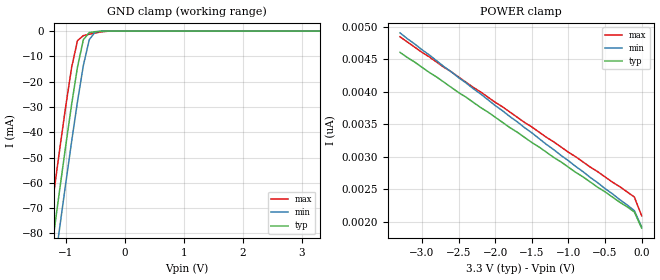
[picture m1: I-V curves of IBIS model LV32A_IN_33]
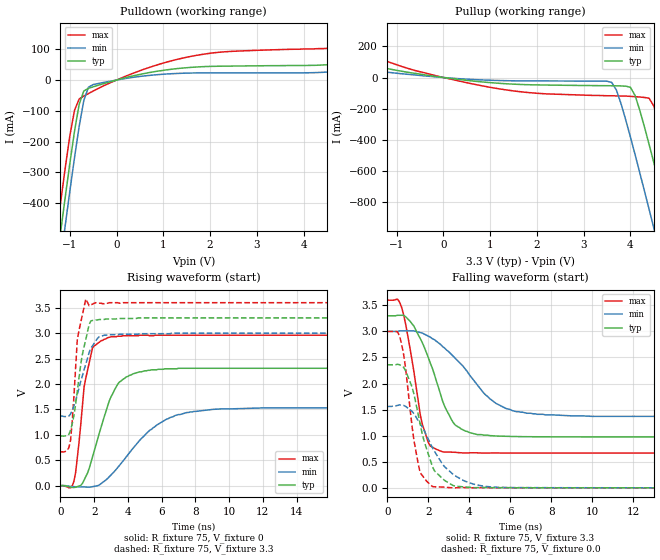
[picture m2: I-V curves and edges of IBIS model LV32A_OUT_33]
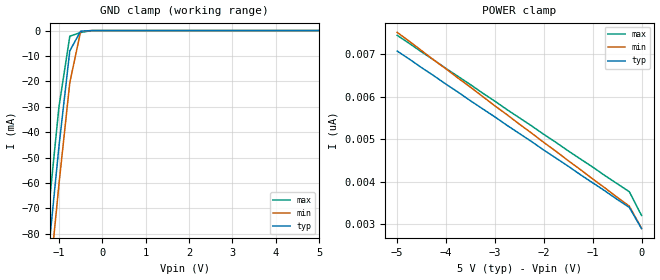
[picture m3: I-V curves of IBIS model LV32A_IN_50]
| TEXAS INSTRUMENTS INCORPORATED
| Standard Linear and Logic Group
| IBIS Model of SN74LV32A
| QUADRUPLE 2-INPUT POSITIVE-NOR GATE
| SOIC 14-pin (D), SOP 14-pin (NS), SSOP 14-pin (DB), TSSOP 14-pin (PW)
| and TVSOP 14-pin (DGV) Package
[IBIS Ver]   3.2
[Comment Char]  |_char
[File Name]   lv32a.ibs
[File Rev]   2.0 H_die
[Date]   May 26, 2000
[Source]   Data created from HSPICE simulations at TI-SLL.
[Notes]   The following is an IBIS list for the LV32A.
|   Please contact sllibis@ti.com with questions and
|   comments concerning SLL IBIS models.
|   The warning about AC Rising Endpoint might be reported,
|   but it is due to HSPICE issue and negligible.
[Disclaimer] Property of Texas Instruments Incorporated.  Unauthorized
   reproduction and/or distribution is strictly prohibited.
   This product is protected under copyright law.
   Created 2000, (C) Copyright 2000, Texas Instruments Inc.,
   All Rights Reserved.
   UNLESS THERE IS A SIGNED, WRITTEN AGREEMENT TO THE
   CONTRARY, TEXAS INSTRUMENTS () IS PROVIDING THE IBIS
   MODELS  AND WITHOUT ANY WARRANTY, EXPRESSED OR
   IMPLIED.  TI assumes no liability for:
   1) the accuracy of the IBIS models provided to your
   company;
   2) the proper functioning of these IBIS Models in your
   design or for any resulting applications; or
   3) infringement of patents, copyrights or intellectual
   property rights resulting from your use of these IBIS
   models.
   TI provides IBIS Models as a service to our customers.
   You and your company shall not distribute, sell or give
   these models to anyone else without prior written
   permission from TI.
   TI reserves the right to make changes to our products or
   to discontinue any semiconductor product or service
   without notice, and advises our customers to obtain the
   latest version of relevant information to verify, before
   placing orders, that the information being relied on is
   current.
   Please be aware that your receipt and use of the IBIS
   information provided shall serve as acceptance of these
   terms and conditions.  If you do not accept these terms,
   you should return or destroy the IBIS models and any
   other accompanying information immediately.
|   Component LV32A_D
[Component]   LV32A_D
[Manufacturer]  Texas Instruments, Inc.
[Package]
|   typ   min   max
R_pkg   0.031   0.028   0.034
L_pkg   3.109nH   2.462nH   3.889nH
C_pkg   0.473pF   0.363pF   0.628pF
[Pin]   signal_name   model_name   R_pin   L_pin   C_pin
1   1A   LV32A_IN   0.033   3.854nH   0.622pF
2   1B   LV32A_IN   0.032   3.188nH   0.473pF
3   1Y   LV32A_OUT   0.028   2.462nH   0.377pF
4   2A   LV32A_IN   0.031   2.596nH   0.363pF
5   2B   LV32A_IN   0.028   2.521nH   0.372pF
6   2Y   LV32A_OUT   0.034   3.250nH   0.476pF
7   GND   GND   0.034   3.889nH   0.628pF
8   3Y   LV32A_OUT   0.034   3.889nH   0.628pF
9   3A   LV32A_IN   0.034   3.250nH   0.476pF
10   3B   LV32A_IN   0.028   2.521nH   0.372pF
11   4Y   LV32A_OUT   0.031   2.596nH   0.364pF
12   4A   LV32A_IN   0.028   2.462nH   0.377pF
13   4B   LV32A_IN   0.032   3.188nH   0.473pF
14   VCC   POWER   0.033   3.854nH   0.622pF
|   Component LV32A_NS
[Component]   LV32A_NS
[Manufacturer]  Texas Instruments, Inc.
[Package]
|   typ   min   max
R_pkg   0.045   0.039   0.054
L_pkg   3.796nH   2.561nH   4.952nH
C_pkg   0.528pF   0.288pF   0.710pF
[Pin]   signal_name   model_name   R_pin   L_pin   C_pin
1   1A   LV32A_IN   0.047   4.867nH   0.706pF
2   1B   LV32A_IN   0.051   4.083nH   0.592pF
3   1Y   LV32A_OUT   0.041   2.915nH   0.376pF
4   2A   LV32A_IN   0.039   2.561nH   0.288pF
5   2B   LV32A_IN   0.041   3.101nH   0.430pF
6   2Y   LV32A_OUT   0.047   4.047nH   0.589pF
7   GND   GND   0.051   4.909nH   0.700pF
8   3Y   LV32A_OUT   0.045   4.784nH   0.694pF
9   3A   LV32A_IN   0.054   4.176nH   0.597pF
10   3B   LV32A_IN   0.039   3.287nH   0.449pF
11   4Y   LV32A_OUT   0.039   2.586nH   0.294pF
12   4A   LV32A_IN   0.040   2.802nH   0.371pF
13   4B   LV32A_IN   0.049   4.080nH   0.593pF
14   VCC   POWER   0.052   4.952nH   0.710pF
|   Component LV32A_DB
[Component]   LV32A_DB
[Manufacturer]  Texas Instruments, Inc.
[Package]
|   typ   min   max
R_pkg   0.044   0.041   0.046
L_pkg   3.551nH   3.258nH   3.927nH
C_pkg   0.402pF   0.360pF   0.421pF
[Pin]   signal_name   model_name   R_pin   L_pin   C_pin
1   1A   LV32A_IN   0.046   3.927nH   0.408pF
2   1B   LV32A_IN   0.044   3.587nH   0.421pF
3   1Y   LV32A_OUT   0.041   3.289nH   0.398pF
4   2A   LV32A_IN   0.042   3.258nH   0.360pF
5   2B   LV32A_IN   0.041   3.286nH   0.403pF
6   2Y   LV32A_OUT   0.044   3.586nH   0.421pF
7   GND   GND   0.046   3.927nH   0.408pF
8   3Y   LV32A_OUT   0.046   3.927nH   0.408pF
9   3A   LV32A_IN   0.044   3.586nH   0.421pF
10   3B   LV32A_IN   0.041   3.286nH   0.403pF
11   4Y   LV32A_OUT   0.043   3.258nH   0.360pF
12   4A   LV32A_IN   0.041   3.289nH   0.398pF
13   4B   LV32A_IN   0.044   3.587nH   0.421pF
14   VCC   POWER   0.046   3.927nH   0.408pF
|   Component LV32A_PW
[Component]   LV32A_PW
[Manufacturer]  Texas Instruments, Inc.
[Package]
|   typ   min   max
R_pkg   0.032   0.029   0.035
L_pkg   2.378nH   2.170nH   2.680nH
C_pkg   0.314pF   0.270pF   0.335pF
[Pin]   signal_name   model_name   R_pin   L_pin   C_pin
1   1A   LV32A_IN   0.033   2.618nH   0.330pF
2   1B   LV32A_IN   0.031   2.313nH   0.317pF
3   1Y   LV32A_OUT   0.030   2.310nH   0.314pF
4   2A   LV32A_IN   0.031   2.173nH   0.272pF
5   2B   LV32A_IN   0.030   2.204nH   0.309pF
6   2Y   LV32A_OUT   0.032   2.315nH   0.317pF
7   GND   GND   0.035   2.680nH   0.335pF
8   3Y   LV32A_OUT   0.033   2.640nH   0.333pF
9   3A   LV32A_IN   0.034   2.347nH   0.319pF
10   3B   LV32A_IN   0.029   2.277nH   0.313pF
11   4Y   LV32A_OUT   0.031   2.170nH   0.270pF
12   4A   LV32A_IN   0.031   2.244nH   0.311pF
13   4B   LV32A_IN   0.033   2.343nH   0.321pF
14   VCC   POWER   0.035   2.657nH   0.332pF
|   Component LV32A_DGV
[Component]   LV32A_DGV
[Manufacturer]  Texas Instruments, Inc.
[Package]
|   typ   min   max
R_pkg   0.035   0.020   0.045
L_pkg   2.499nH   2.077nH   2.966nH
C_pkg   0.361pF   0.305pF   0.416pF
[Pin]   signal_name   model_name   R_pin   L_pin   C_pin
1   1A   LV32A_IN   0.027   2.717nH   0.373pF
2   1B   LV32A_IN   0.037   2.434nH   0.398pF
3   1Y   LV32A_OUT   0.034   2.200nH   0.316pF
4   2A   LV32A_IN   0.020   2.077nH   0.309pF
5   2B   LV32A_IN   0.030   2.147nH   0.305pF
6   2Y   LV32A_OUT   0.042   2.580nH   0.408pF
7   GND   GND   0.039   2.921nH   0.385pF
8   3Y   LV32A_OUT   0.033   2.841nH   0.380pF
9   3A   LV32A_IN   0.042   2.611nH   0.410pF
10   3B   LV32A_IN   0.038   2.331nH   0.329pF
11   4Y   LV32A_OUT   0.026   2.223nH   0.319pF
12   4A   LV32A_IN   0.034   2.259nH   0.313pF
13   4B   LV32A_IN   0.045   2.681nH   0.416pF
14   VCC   POWER   0.042   2.966nH   0.386pF
[Model Selector]   LV32A_IN
LV32A_IN_33   3.3-V Vcc Input Model
LV32A_IN_50   5.0-V Vcc Input Model
[Model Selector]   LV32A_OUT
LV32A_OUT_33   3.3-V Vcc Output Model
LV32A_OUT_50   5.0-V Vcc Output Model
| Models and submodels in the file (4): LV32A_IN_33 (Input), LV32A_OUT_33 (Output), LV32A_IN_50 (Input), LV32A_OUT_50 (Output)
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|   Model LV32A_IN_33
[Model]   LV32A_IN_33
Model_type  Input
Polarity   Inverting
Vinl = 0.99
Vinh = 2.31
| variable   typ   min   max
C_comp   1.24pf   0.94pf   1.54pf
[Temperature Range]   25   85   -40
[Voltage Range]   3.3   3.0   3.6
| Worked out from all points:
|   GND clamp passes 1 mA (typ) near -0.61 V on its own axis
[GND Clamp]
|   Voltage   I(typ)   I(min)   I(max)
-3.3V     -460mA     -475mA     -445mA
-1.3V     -97.5mA    -113mA     -81.5mA
-1.2V     -79.9mA    -95mA      -63.9mA
-1.1V     -62.6mA    -77.6mA    -46.7mA
-1V       -45.6mA    -60.5mA    -30mA
-900mV    -29.2mA    -43.9mA    -14.6mA
-800mV    -14.3mA    -28mA      -3.81mA
-700mV    -3.42mA    -13.6mA    -1.78mA
-600mV    -581uA     -3.4mA     -1.25mA
-500mV    -233uA     -353uA     -759uA
-400mV    -58.1uA    -21.9uA    -324uA
3.3V      1.9nA      2.34nA     1.69nA
[POWER Clamp]
|   Voltage   I(typ)   I(min)   I(max)
-3.3V     4.61nA     4.91nA     4.85nA
-3V       4.38nA     4.65nA     4.61nA
-100mV    2.15nA     2.17nA     2.38nA
0V        1.9nA      1.92nA     2.09nA
|   Model LV32A_OUT_33
[Model]   LV32A_OUT_33
Model_type  Output
Polarity   Non-Inverting
Vmeas = 1.65v
Cref = 15pf
| variable   typ   min   max
C_comp   4.62pf   3.47pf   5.77pf
[Temperature Range]   25   85   -40
[Voltage Range]   3.3   3.0   3.6
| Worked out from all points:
|   slope of the pulldown table from 0 to 0.495 V, typ, clamps not added: 27.3 ohm
|   slope of the pullup table from 0 to 0.495 V, typ, clamps not added: 27.2 ohm
|   rising waveform, R_fixture 75, V_fixture 0: 20-80 % time 1.34ns typ, 2.6ns min, 659ps max; typ from 0 V to 2.31 V
|   falling waveform, R_fixture 75, V_fixture 3.3: 20-80 % time 1.31ns typ, 2.23ns min, 735ps max; typ from 3.3 V to 0.976 V
|   rising waveform, R_fixture 75, V_fixture 3.3: 20-80 % time 648ps typ, 847ps min, 383ps max; typ from 0.976 V to 3.3 V
|   falling waveform, R_fixture 75, V_fixture 0.0: 20-80 % time 908ps typ, 1.48ns min, 589ps max; typ from 2.36 V to 0 V
[Pulldown]
|   Voltage   I(typ)   I(min)   I(max)
-3.3V     -3.04A     -3.13A     -2.95A
-1.3V     -615mA     -707mA     -518mA
-1.2V     -498mA     -591mA     -401mA
-1.1V     -383mA     -475mA     -288mA
-900mV    -167mA     -253mA     -98.6mA
-800mV    -79.1mA    -151mA     -61.7mA
-700mV    -35.5mA    -66.4mA    -51.9mA
-600mV    -26.8mA    -23.2mA    -43.9mA
-500mV    -22mA      -14.7mA    -35.8mA
1.6V      41.2mA     22.8mA     77.1mA
4.7V      52.1mA     27.5mA     106mA
6.6V      86.8mA     47.3mA     166mA
[Pullup]
|   Voltage   I(typ)   I(min)   I(max)
-3.3V     166mA      91.1mA     311mA
600mV     -21.6mA    -12.3mA    -39.7mA
3.6V      -52.9mA    -31.5mA    -117mA
3.8V      -54.2mA    -168mA     -119mA
4V        -62.6mA    -381mA     -121mA
4.1V      -115mA     -494mA     -123mA
4.4V      -429mA     -845mA     -133mA
4.5V      -544mA     -964mA     -182mA
4.8V      -899mA     -1.32A     -505mA
4.9V      -1.02A     -1.44A     -622mA
5.2V      -1.38A     -1.81A     -981mA
6.6V      -3.09A     -3.52A     -2.69A
[Ramp]
| variable   typ   min   max
dV/dt_r   1.40E+00/1.34E-09   9.37E-01/2.69E-09   1.78E+00/5.83E-10
dV/dt_f   1.41E+00/1.29E-09   9.88E-01/2.24E-09   1.77E+00/7.57E-10
R_load = 75
[Rising Waveform]
R_fixture = 75
V_fixture = 0
|   Time   V(typ)   V(min)   V(max)
0s        0V         0V         0V
800ps     -35.5mV    -19.6mV    87.5mV
1.1ns     -7.6mV     -22.7mV    848mV
1.4ns     110mV      -25.5mV    1.94V
1.9ns     564mV      -19.7mV    2.71V
2.8ns     1.57V      143mV      2.91V
3.9ns     2.14V      565mV      2.95V
5.7ns     2.28V      1.19V      2.96V
7.5ns     2.31V      1.44V      2.96V
25ns      2.31V      1.53V      2.96V
[Falling Waveform]
R_fixture = 75
V_fixture = 3.3
V_fixture_min = 3.0
V_fixture_max = 3.6
|   Time   V(typ)   V(min)   V(max)
0s        3.3V       3V         3.6V
700ps     3.31V      3.01V      3.46V
1.7ns     2.79V      2.97V      1.23V
2.1ns     2.39V      2.89V      799mV
2.7ns     1.66V      2.71V      689mV
3.2ns     1.26V      2.53V      683mV
3.8ns     1.09V      2.28V      668mV
5ns       1V         1.71V      667mV
6.3ns     983mV      1.46V      667mV
25ns      976mV      1.37V      666mV
[Rising Waveform]
R_fixture = 75
V_fixture = 3.3
V_fixture_min = 3.0
V_fixture_max = 3.6
|   Time   V(typ)   V(min)   V(max)
0s        976mV      1.37V      666mV
400ps     985mV      1.36V      694mV
600ps     1.09V      1.41V      893mV
800ps     1.38V      1.57V      1.76V
1ns       1.86V      1.8V       2.88V
1.2ns     2.38V      2.05V      3.21V
1.5ns     2.87V      2.39V      3.67V
1.8ns     3.24V      2.7V       3.56V
2.8ns     3.28V      2.97V      3.59V
25ns      3.3V       3V         3.6V
[Falling Waveform]
R_fixture = 75
V_fixture = 0.0
|   Time   V(typ)   V(min)   V(max)
0s        2.36V      1.56V      3V
600ps     2.36V      1.59V      2.91V
800ps     2.31V      1.58V      2.55V
900ps     2.24V      1.56V      2.27V
1.2ns     1.94V      1.47V      1.2V
1.6ns     1.23V      1.23V      291mV
2.2ns     406mV      770mV      23.3mV
3.2ns     45mV       260mV      -1.64mV
4.8ns     4.61mV     25.3mV     2.29mV
25ns      11.1uV     556nV      13.7uV
|   Model LV32A_IN_50
[Model]   LV32A_IN_50
Model_type  Input
Polarity   Inverting
Vinl = 1.5
Vinh = 3.5
| variable   typ   min   max
C_comp   1.24pf   0.94pf   1.54pf
[Temperature Range]   25   85   -40
[Voltage Range]   5.0   4.5   5.5
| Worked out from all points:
|   GND clamp passes 1 mA (typ) near -0.52 V on its own axis
[GND Clamp]
|   Voltage   I(typ)   I(min)   I(max)
-5V       -773mA     -786mA     -758mA
-1.5V     -133mA     -148mA     -117mA
-1.25V    -88.7mA    -104mA     -72.7mA
-1V       -45.6mA    -60.5mA    -30mA
-750mV    -7.99mA    -20.5mA    -2.23mA
-500mV    -233uA     -353uA     -759uA
-250mV    -2.63nA    -182nA     -26.9uA
5V        2.9nA      3.64nA     2.54nA
[POWER Clamp]
|   Voltage   I(typ)   I(min)   I(max)
-5V       7.08nA     7.52nA     7.45nA
-1.5V     4.37nA     4.5nA      4.73nA
-250mV    3.4nA      3.43nA     3.77nA
0V        2.9nA      2.91nA     3.21nA
